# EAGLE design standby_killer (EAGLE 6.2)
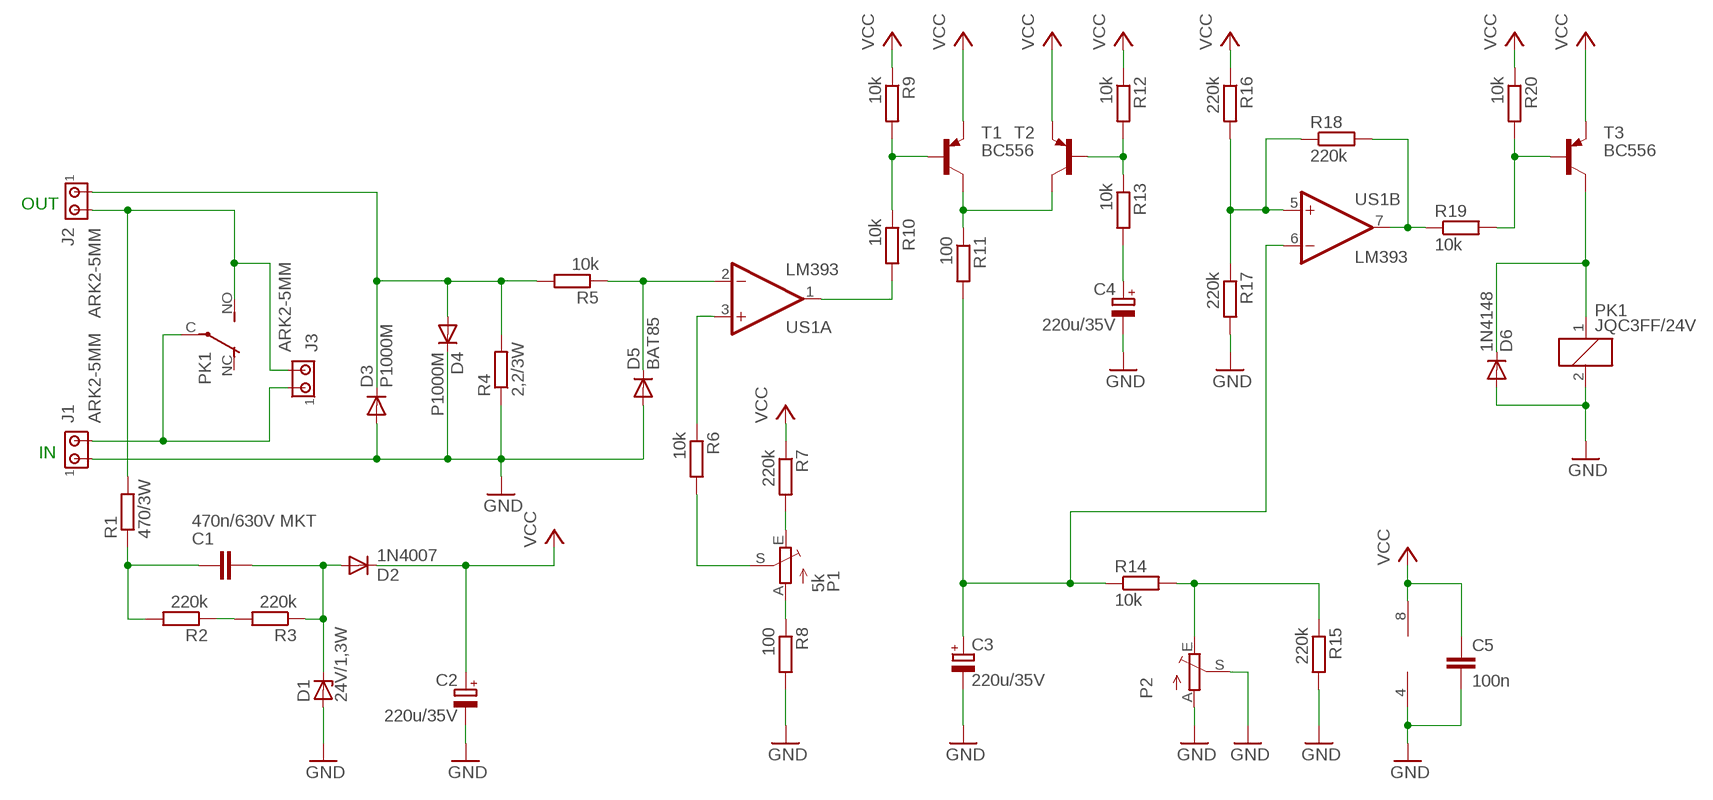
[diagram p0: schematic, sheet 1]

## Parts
C1  470n/630V MKT  C-EU225-108X268  [C225-108X268]
C2  220u/35V  CPOL-EUE3.5-8  [E3,5-8]
C3  220u/35V  CPOL-EUE3.5-8  [E3,5-8]
C4  220u/35V  CPOL-EUE3.5-8  [E3,5-8]
C5  100n  C-EU050-025X075  [C050-025X075]
D1  24V/1,3W  ZENER-DIODEDO41Z10  [DO41Z10]
D2  1N4007  1N4004  [DO41-10]
D3  P1000M  DIODE-P6-15  [P6-15]
D4  P1000M  DIODE-P6-15  [P6-15]
D5  BAT85  1N4148DO35-7  [DO35-7]
D6  1N4148  1N4148DO35-7  [DO35-7]
J1  ARK2-5MM  [2PIN-5MM]
J2  ARK2-5MM  [2PIN-5MM]
J3  ARK2-5MM  [2PIN-5MM]
P1  5k  TRIM_EU-CA6V  [CA6V]
P2  TRIM_EU-CA6V  [CA6V]
PK1  JQC3FF/24V  PK_POJED-JQC-3FG  [PK_POJED_JQC-3FG]
R1  470/3W  R-EU_0617/17  [0617/17]
R2  220k  R-EU_0207/7  [0207/7]
R3  220k  R-EU_0207/7  [0207/7]
R4  2,2/3W  R-EU_0617/17  [0617/17]
R5  10k  R-EU_0207/15  [0207/15]
R6  10k  R-EU_0207/7  [0207/7]
R7  220k  R-EU_0207/7  [0207/7]
R8  100  R-EU_0207/7  [0207/7]
R9  10k  R-EU_0204/2V  [0204V]
R10  10k  R-EU_0207/7  [0207/7]
R11  100  R-EU_0207/7  [0207/7]
R12  10k  R-EU_0204/2V  [0204V]
R13  10k  R-EU_0207/7  [0207/7]
R14  10k  R-EU_0207/7  [0207/7]
R15  220k  R-EU_0207/7  [0207/7]
R16  220k  R-EU_0207/7  [0207/7]
R17  220k  R-EU_0207/7  [0207/7]
R18  220k  R-EU_0207/7  [0207/7]
R19  10k  R-EU_0207/7  [0207/7]
R20  10k  R-EU_0207/7  [0207/7]
T1  BC556  [TO92-EBC]
T2  BC556  [TO92-EBC]
T3  BC556  [TO92-EBC]
US1  LM393  LM393N  [DIL08]

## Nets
GND: C2.- C3.- C4.- C5.2 D1.A D3.A D4.C D5.A D6.A J1.P$1 P2.A P2.S PK1.2 R4.1 R8.2 R15.2 R17.2 US1.4(P:V-)
N$1: D3.C D4.A J2.P$1 R4.2 R5.2
N$2: R10.2 US1.1(A:OUT)
N$3: D5.C R5.1 US1.2(A:-IN)
N$4: R6.1 US1.3(A:+IN)
N$6: P1.A R8.1
N$7: P1.E R7.2
N$8: P1.S R6.2
N$9: R9.2 R10.1 T1.B
N$10: R11.1 T1.C T2.C
N$11: R12.2 R13.1 T2.B
N$12: C3.+ R11.2 R14.1 US1.6(B:-IN)
N$13: R16.2 R17.1 R18.1 US1.5(B:+IN)
N$14: R18.2 R19.1 US1.7(B:OUT)
N$15: D6.C PK1.1 T3.C
N$16: J1.P$2 J3.P$1 PK1.C(COM)
N$17: R19.2 R20.2 T3.B
N$18: J2.P$2 J3.P$2 PK1.NO R1.2
N$19: C1.2 D1.C D2.A R3.1
N$20: R2.1 R3.2
N$21: C1.1 R1.1 R2.2
N$22: P2.E R14.2 R15.1
N$23: C4.+ R13.2
VCC: C2.+ C5.1 D2.C R7.1 R9.1 R12.1 R16.1 R20.1 T1.E T2.E T3.E US1.8(P:V+)
Unconnected: PK1.NC

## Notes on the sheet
- OUT
- IN

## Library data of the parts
C1 C5 = rcl:C-EU: CAPACITOR, European symbol
C2-C4 = rcl:CPOL-EU: POLARIZED CAPACITOR, European symbol
D1 = diode:ZENER-DIODE: Z-Diode
D2 = diode:1N4004: DIODE
D3 D4 = diode:DIODE-: DIODE
D5 D6 = diode:1N4148: DIODE
J1-J3 = zlacza_futrzak:ARK2: ARK 2
P1 P2 = pot:TRIM_EU-: POTENTIOMETER
PK1 = inne_futrzak:PK_POJED
R1-R20 = rcl:R-EU_: RESISTOR, European symbol
T1-T3 = transistor-pnp:BC556*: PNP Transistror
US1 = linear:LM393: COMPARATOR

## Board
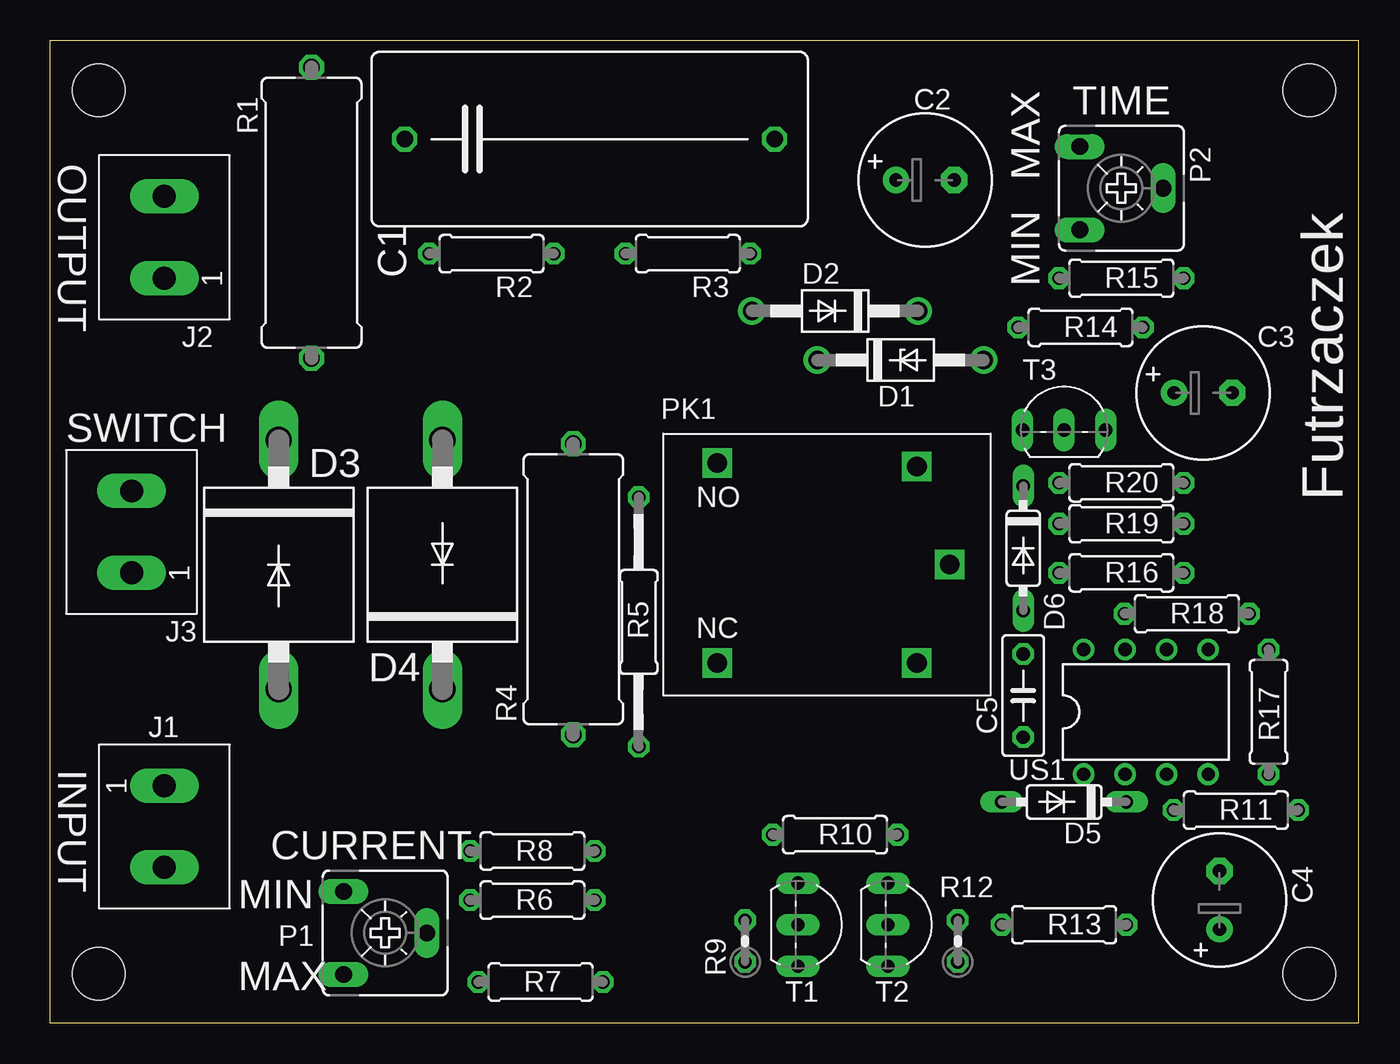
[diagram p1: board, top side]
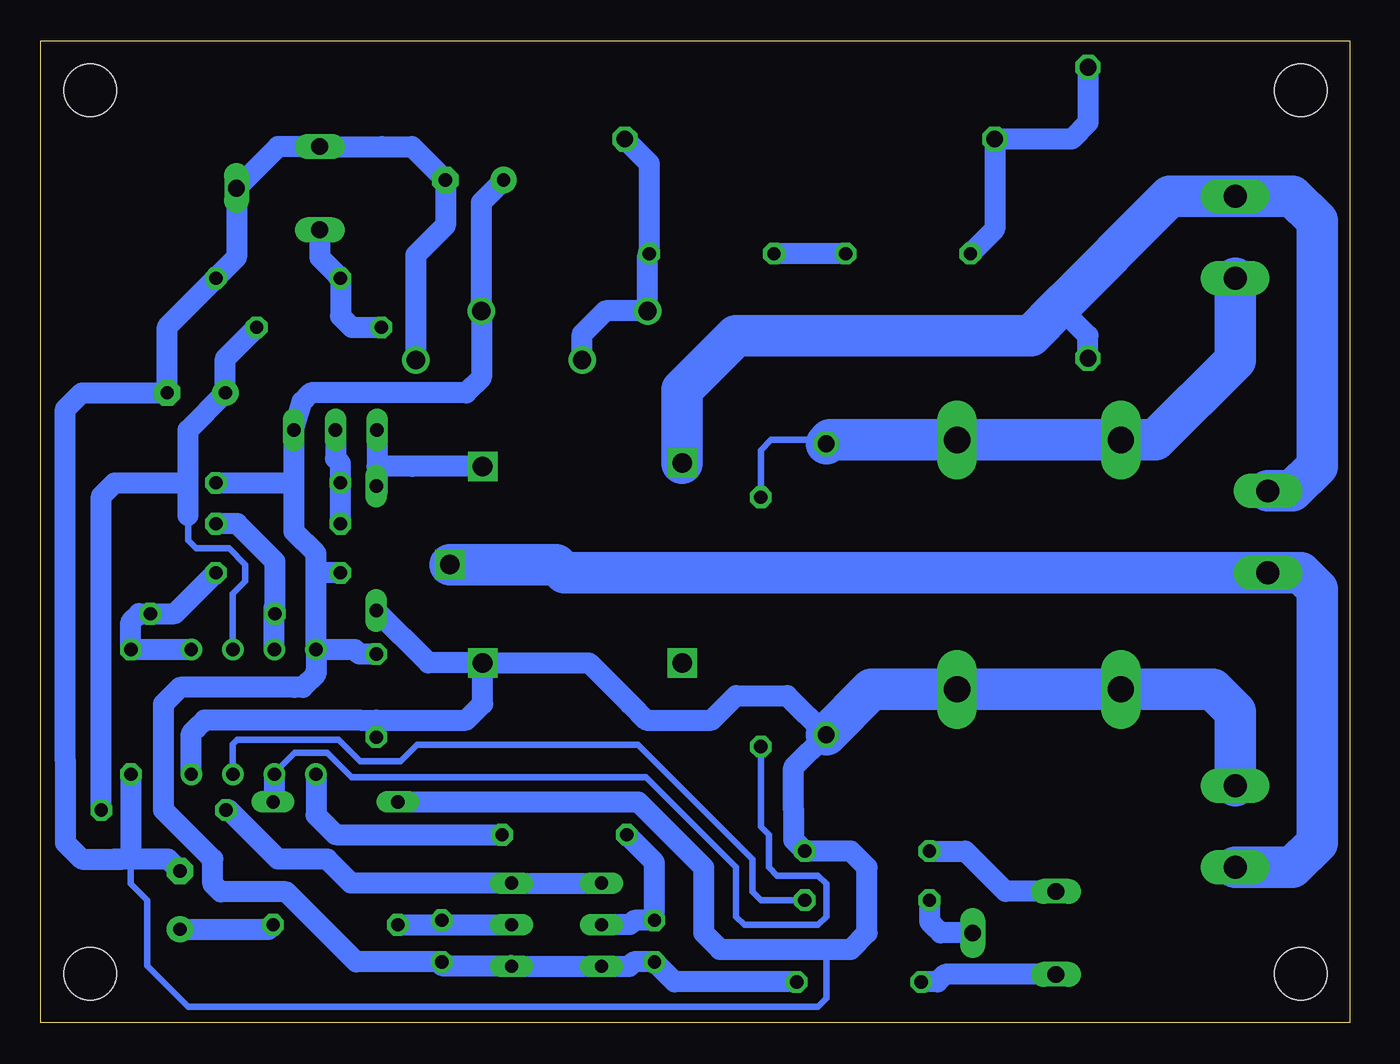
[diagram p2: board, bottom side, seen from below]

Size 80 x 60 mm. Coordinates in mm from the lower left corner, seen from the top.
Outline: 0,0 80,0 80,60 0,60 0,0
Copper layers (1*16): Top 0.035mm / dielectric 1.5mm / Bottom 0.035mm
Design rules: minimum track width 10mil, minimum drill 23mil, track to track 8mil, track to pad 8mil, pad to pad 8mil, via to via 8mil, smd to smd 8mil, copper to edge 20mil, drill to drill 8mil, minimum pad ring 10mil, minimum via ring 8mil, stop-mask expansion 4mil, vias tented up to drill 0mil, thermal gap 10mil
Holes 3.2 mm at 3,3 3,57 77,3 77,57

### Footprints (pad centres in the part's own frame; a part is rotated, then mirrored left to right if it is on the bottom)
C225-108X268 = drill 1.016 octagon: 1 -11.303,0; 2 11.303,0
E3,5-8 = drill 0.813 pad 1.6: + -1.778,0 | drill 0.813 pad 1.6 octagon: - 1.778,0
C050-025X075 = drill 0.813 octagon: 1 -2.54,0; 2 2.54,0
DO41Z10 = drill 1.118: A 5.08,0; C -5.08,0
DO41-10 = drill 1.118: A 5.08,0; C -5.08,0
P6-15 = drill 1.6 long: A 7.62,0; C -7.62,0
DO35-7 = drill 0.813 long: A 3.81,0; C -3.81,0
2PIN-5MM = drill 1.4 long: P$1 -2.5,0; P$2 2.5,0
CA6V = drill 1.016 long: A -2.54,-2.54; E 2.54,-2.54; S 0,2.54
PK_POJED_JQC-3FG = drill 1.2 square: 1 5.5,6; 2 5.5,-6; C 7.5,0; NC -6.7,-6; NO -6.7,6.2
0617/17 = drill 1.016 octagon: 1 -8.89,0; 2 8.89,0
0207/7 = drill 0.813 octagon: 1 -3.81,0; 2 3.81,0
0207/15 = drill 0.813 octagon: 1 -7.62,0; 2 7.62,0
0204V = drill 0.813 octagon: 1 -1.27,0; 2 1.27,0
TO92-EBC = drill 0.813 long: B 0,-1.27; C -2.54,-1.27; E 2.54,-1.27
DIL08 = drill 0.813 pad 1.27: 1 -3.81,-3.81; 2 -1.27,-3.81; 3 1.27,-3.81; 4 3.81,-3.81; 5 3.81,3.81; 6 1.27,3.81; 7 -1.27,3.81; 8 -3.81,3.81

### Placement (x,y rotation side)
C1  33,54 0 top
C2  53.5,51.5 0 top
C3  70.5,38.5 0 top
C4  71.5,7.5 90 top
C5  59.5,20 270 top
D1  52,40.5 0 top
D2  48,43.5 180 top
D3  14,28 270 top
D4  24,28 90 top
D5  62,13.5 180 top
D6  59.5,29 270 top
J1  7,12 270 top
J2  7,48 90 top
J3  5,30 90 top
P1  20.5,5.5 270 top
P2  65.5,51 270 top
PK1  47.5,28 0 top
R1  16,49.5 270 top
R2  27,47 180 top
R3  39,47 180 top
R4  32,26.5 90 top
R5  36,24.5 90 top
R6  29.5,7.5 180 top
R7  30,2.5 180 top
R8  29.5,10.5 0 top
R9  42.5,5 90 top
R10  48,11.5 0 top
R11  72.5,13 0 top
R12  55.5,5 90 top
R13  62,6 0 top
R14  63,42.5 180 top
R15  65.5,45.5 0 top
R16  65.5,27.5 0 top
R17  74.5,19 270 top
R18  69.5,25 180 top
R19  65.5,30.5 180 top
R20  65.5,33 180 top
T1  47,6 270 top
T2  52.5,6 270 top
T3  62,37.5 0 top
US1  67,19 0 top

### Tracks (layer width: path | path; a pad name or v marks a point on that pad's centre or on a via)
GND
  Bottom 0.406: 32,4.5 32,1.5 32.5,1 44,1 71,1 73.5,3.5 73.5,5.5 73.5,7.5 74.5,8.5 74.5,10
  Bottom 1.27: D5.A 54.5,13.5 43.5,13.5 39.5,9.5 39.5,5.5 38.5,4.5 32,4.5 30.5,4.5 29.5,5.5 29.5,9.5 30.5,10.5 R8.2 34,11.19 34,13 34,15.61 R4.1 34.39,20 37.5,20 39,18.5 43,18.5 44,19.5 46.5,22 PK1.2 | R17.2 74.5,12.28 74.5,10 | 75.5,10 77.5,10 78.5,11 78.5,16 78.5,37.5 77.5,38.5 C3.- 72.28,42.53 R15.2 68.04,46.77 P2.S 65.5,53.54 P2.A 59.16,53.54 57.32,53.54 C2.- 55.28,48.72 56,48 57.08,46.92 D1.A | 75.5,10 75,10 74.5,10 | C4.- 72.22,10 74.5,10 | 74.5,10 75.5,10 | PK1.2 56.31,22 D6.A | 59.5,18.5 60.5,18.5 67.5,18.5 70,18.5 70.5,18 70.81,17.69 US1.4 | 59.5,18.5 54,18.5 53,19.5 PK1.2 | 59.5,18.5 59.5,17.5 C5.2
  Bottom 2.54: J1.P$1 7,19 8.38,20.38 D3.A D4.C 29.23,20.38 R4.1
N$1
  Bottom 0.406: 32.23,35.62 35.38,35.62 36,35 R5.2
  Bottom 1.27: 32.23,35.62 R4.2
  Bottom 2.54: J2.P$1 7,40.5 11.88,35.62 D3.C D4.A 30.73,35.62 | 30.73,35.62 31.77,35.62 | 31.77,35.62 30.73,35.62 | 30.73,35.62 31.77,35.62 | 31.77,35.62 R4.2
N$2
  Bottom 1.27: US1.1 63.19,12.69 62,11.5 R10.2
N$3
  Bottom 0.406: US1.2 65.73,15.27 65,16 64.5,16.5 62.5,16.5 61,15 57.5,15 43,15 40,12 37.5,9.5 37.5,6.5 37,6 32.5,6 32,6.5 32,8.5 32.5,9 35,9 35.5,9.5 35.5,11.5 36,12 R5.1
  Bottom 1.27: US1.2 65.73,13.58 D5.C
N$4
  Bottom 0.406: US1.3 68.27,17.03 68,17.3 61.8,17.3 60.5,16 58,16 57,17 43.5,17 39,12.5 36.5,10 36.5,8 36,7.5 R6.1
N$6
  Bottom 1.27: R8.1 23.5,10.5 21.5,8.5 21.04,8.04 P1.A
N$7
  Bottom 1.27: P1.E 24.73,2.96 25.19,2.5 R7.2
N$8
  Bottom 1.27: P1.S 25,5.5 25.5,6 25.69,6.19 R6.2
N$9
  Bottom 1.27: T1.B 44,6 43.73,6.27 R9.2 42.5,9.81 R10.1
N$10
  Bottom 1.27: T1.C T2.C 61.04,8.54 62.5,10 65.5,10 68.5,13 R11.1
N$11
  Bottom 1.27: R13.1 55.5,6 | 55.5,6 T2.B | R12.2 55.5,6
N$12
  Bottom 0.406: US1.6 68.27,26.23 67.5,27 67.5,28 68.5,29 70.5,29 71,29.5 71,31
  Bottom 1.27: R14.1 68.72,40.59 C3.+ 71,36.22 71,35 | 71,31 71,33 | 71,33 71,35 | 71,34.81 71,35 | R11.2 76.31,32.19 75.5,33 71,33
N$13
  Bottom 1.27: US1.5 R17.1 74.5,24.5 74,25 R18.1 71.81,25 R16.2
N$14
  Bottom 1.27: US1.7 65.73,25.46 R18.2 65.69,28.19 68,30.5 R19.1
N$15
  Bottom 1.27: PK1.1 57.31,34 59.46,34 | T3.C 59.46,34 | 59.46,34 59.46,32.35 D6.C
N$16
  Bottom 2.54: J1.P$2 3.5,9.5 2,11 2,26.5 3,27.5 J3.P$1 48,27.5 48.5,28 PK1.C
N$17
  Bottom 1.27: T3.B 62,34.5 61.69,34.19 R20.2 R19.2
N$18
  Bottom 1.27: R1.2 16,42 17.75,43.75
  Bottom 2.54: J3.P$2 3.5,32.5 2,34 2,49 3.5,50.5 J2.P$2 11,50.5 12,49.5 17,44.5 17.75,43.75 19.5,42 33,42 37.5,42 39,40.5 40.8,38.7 PK1.NO
N$19
  Bottom 1.27: C1.2 42.81,52.51 R3.1 42.92,46.89 D2.A 45.5,43.5 46.5,42.5 46.92,42.08 D1.C
N$20
  Bottom 1.27: R2.1 R3.2
N$21
  Bottom 1.27: R1.1 16,55 17,54 C1.1 21.7,48.49 R2.2
N$22
  Bottom 1.27: P2.E 62.96,46.77 R15.1 61.69,43.19 61,42.5 R14.2
N$23
  Bottom 1.27: C4.+ 66.09,5.72 R13.2
VCC
  Bottom 1.27: 64.54,33 T3.E 64.04,37.96 63.5,38.5 54,38.5 53.08,39.42 D2.C 53.08,50.14 C2.+ | 64.54,33 64.54,30.04 63.19,28.69 63.19,27.5 | R20.1 64.54,33 | US1.8 63.19,27.5 | R16.1 63.19,27.5 | US1.8 63.19,21.5 63.19,21.31 64,20.5 64.5,20.5 71.5,20.5 72.5,19.5 72.5,13 69.5,10 69.5,8.5 69,8 65,8 64.5,7.5 60.73,3.73 R12.1 55.5,3.5 51.27,3.5 T2.E T1.E 44.04,3.46 44,3.5 43.77,3.73 R9.1 41.27,2.5 R7.1 | C5.1 60.54,22.54 60.81,22.81 US1.8

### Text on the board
tPlace: TIME | OUTPUT | MAX | Futrzaczek | MIN | SWITCH | INPUT | CURRENT | MIN | MAX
